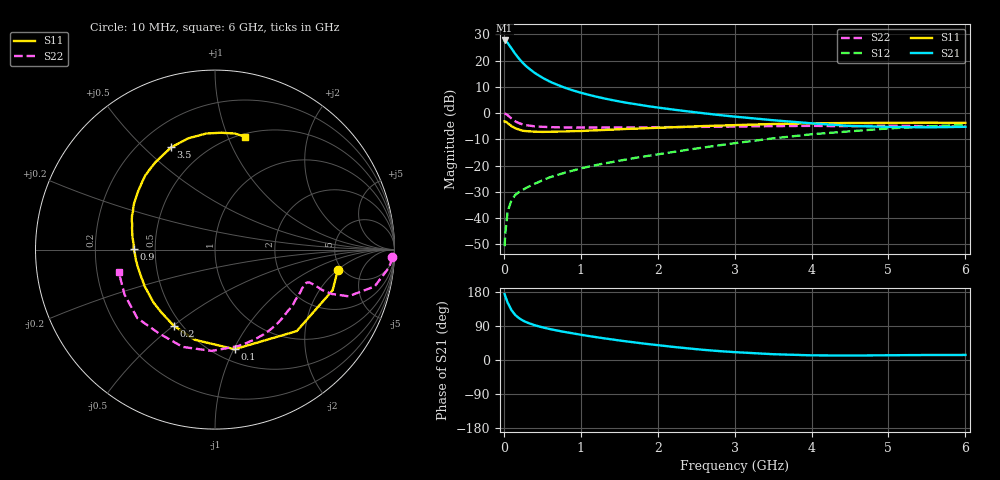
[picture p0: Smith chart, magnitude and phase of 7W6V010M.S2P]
! Infineon Technologies  Discrete & RF Semiconductors
! BFS17W
! Si NPN RF Bipolar Junction Transistor in SOT323
! VCE = 6 V  IC = 10 mA
! Common Emitter S-Parameters:  August  1999
# GHz  S  MA  R  50
!  f  S11  S21  S12  S22
! GHz  MAG  ANG  MAG  ANG  MAG  ANG  MAG  ANG
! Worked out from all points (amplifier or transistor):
!   36 points, 10 MHz to 6 GHz, reference 50 ohm
!   highest |S21| = 27.7 dB at 10 MHz (marker M1)
!   |S21| within 3 dB of that: start of sweep to 98.65 MHz
!   unconditionally stable (mu >= 1): 414.5 MHz to 2.265 GHz; 5.267 GHz to end of sweep
!   at 250 MHz: K = 0.79, MSG = 24.1 dB, |S12| = -29.2 dB
!   at 1.4 GHz: K = 1.18, MAG = 9.3 dB, |S12| = -18.7 dB
!   at 6 GHz: K = 1.05, MAG = -1.7 dB, |S12| = -4.5 dB
!   S11 on the Smith chart (normalised r, x): 10 MHz: 4.63, -2.00; 100 MHz: 0.62, -1.01; 200 MHz: 0.45, -0.50; 900 MHz: 0.38, +0.01; 3.5 GHz: 0.33, +0.61; 6 GHz: 0.53, +1.16
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0.01  0.6937 -9.3  24.3 174.0  0.0029 80.5  0.9897 -2.5
0.02  0.6934 -19.1  24.05 167.6  0.0053 83.4  0.9752 -5.8
0.05  0.6432 -44.9  21.74 151.2  0.0135 73.5  0.9129 -13.0
0.1  0.5656 -78.9  17.09 131.4  0.022 59.7  0.7875 -19.3
0.15  0.5147 -102.8  13.38 118.4  0.0277 55.2  0.6956 -20.8
0.2  0.4824 -118.5  10.8 110.1  0.0315 55.0  0.6408 -20.7
0.25  0.4605 -130.3  8.945 103.9  0.0345 54.3  0.6061 -20.0
0.3  0.452 -139.3  7.62 99.1  0.0381 56.8  0.5856 -19.6
0.4  0.4419 -152.1  5.86 91.8  0.0448 58.7  0.5597 -19.2
0.5  0.4385 -160.5  4.744 86.3  0.0521 60.9  0.5482 -19.4
0.6  0.4405 -166.9  3.976 81.6  0.0598 62.9  0.5408 -20.1
0.7  0.4443 -172.0  3.441 77.5  0.0664 64.6  0.5361 -21.4
0.9  0.4538 179.3  2.704 70.2  0.0804 66.5  0.5307 -24.4
1.1  0.4639 171.9  2.24 63.3  0.0952 67.5  0.5299 -28.2
1.3  0.4773 165.6  1.913 57.3  0.1096 68.5  0.529 -32.5
1.6  0.5002 157.5  1.572 48.9  0.131 69.5  0.5309 -39.3
2.2  0.5375 142.9  1.168 34.6  0.1812 71.2  0.5417 -54.7
2.8  0.5771 128.7  0.919 23.5  0.2431 70.1  0.5494 -71.3
3.5  0.62 113.2  0.732 15.3  0.33 65.6  0.5648 -91.8
4.5  0.6486 94.3  0.57 11.7  0.4498 53.5  0.5615 -124.0
5.5  0.6559 80.4  0.536 13.2  0.5563 40.4  0.5628 -153.7
6  0.6512 75.0  0.548 13.3  0.5982 34.0  0.5507 -166.9
